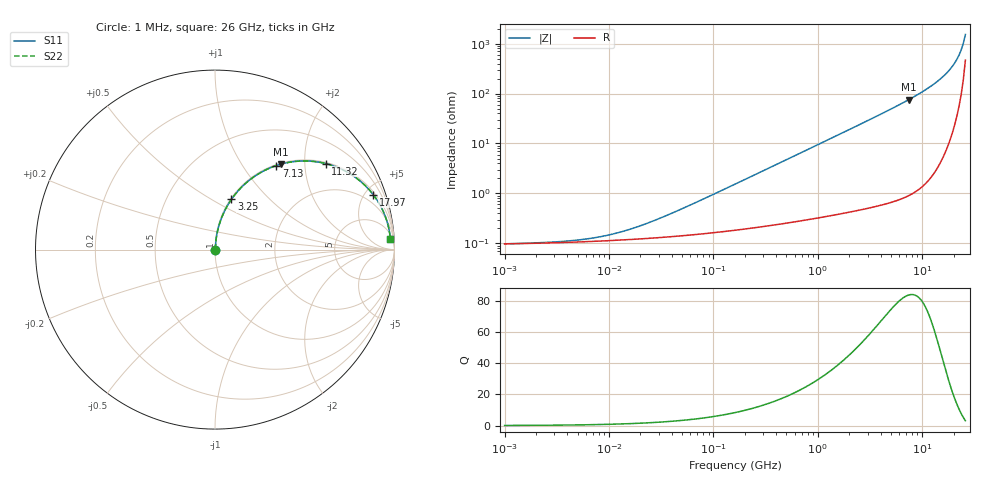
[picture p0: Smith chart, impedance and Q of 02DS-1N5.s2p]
# MHz S MA R 50
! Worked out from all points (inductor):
!   221 points, 1 MHz to 26 GHz, reference 50 ohm
!   read as one part in series: L = 1.5 nH near 44.22 MHz
!   highest Q = 83.7 at 7.467 GHz (marker M1), where L = 1.61 nH
!   S11 on the Smith chart (normalised r, x): 1 MHz: 1.00, +0.00; 3.25 GHz: 1.01, +0.62; 7.13 GHz: 1.02, +1.44; 11.32 GHz: 1.03, +2.54; 17.97 GHz: 1.20, +5.69; 26 GHz: 10, +29
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1  0.0009766 5.5  0.999 -0.0  0.999 -0.0  0.0009766 5.5
2.76374  0.001053 14.3  0.999 -0.0  0.999 -0.0  0.001053 14.3
5.52737  0.00119 25.9  0.9989 -0.0  0.9989 -0.0  0.00119 25.9
8.37782  0.001362 35.3  0.9989 -0.0  0.9989 -0.0  0.001362 35.3
12.6982  0.001665 45.8  0.9988 -0.1  0.9988 -0.1  0.001665 45.8
30.5518  0.003157 65.5  0.9987 -0.2  0.9987 -0.2  0.003157 65.5
168.871  0.01599 82.5  0.998 -0.9  0.998 -0.9  0.01599 82.5
891.261  0.08359 83.1  0.9934 -4.8  0.9934 -4.8  0.08359 83.1
1782.48  0.1657 79.1  0.9822 -9.5  0.9822 -9.5  0.1657 79.1
3250.2  0.2951 71.9  0.9505 -17.2  0.9505 -17.2  0.2951 71.9
4926.33  0.4297 63.8  0.8972 -25.4  0.8972 -25.4  0.4297 63.8
7129.64  0.5798 53.9  0.8078 -35.4  0.8078 -35.4  0.5798 53.9
7466.82  0.6 52.4  0.7929 -36.9  0.7929 -36.9  0.6 52.4
9407.54  0.702 44.7  0.7037 -44.6  0.7037 -44.6  0.702 44.7
11317.4  0.7807 37.9  0.6142 -51.3  0.6142 -51.3  0.7807 37.9
14933.3  0.8828 26.8  0.4517 -62.0  0.4517 -62.0  0.8828 26.8
17965.1  0.9334 19.1  0.3281 -68.9  0.3281 -68.9  0.9334 19.1
20636.4  0.9597 13.3  0.2302 -73.3  0.2302 -73.3  0.9597 13.3
22634.4  0.9711 9.4  0.1635 -75.2  0.1635 -75.2  0.9711 9.4
23704.9  0.9749 7.4  0.13 -75.2  0.13 -75.2  0.9749 7.4
24825.9  0.9774 5.5  0.09669 -73.8  0.09669 -73.8  0.9774 5.5
26000  0.9786 3.5  0.06406 -68.8  0.06406 -68.8  0.9786 3.5
